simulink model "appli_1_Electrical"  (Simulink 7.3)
settings: Solver=ode23t  StartTime=0.0  StopTime=10.0  RelTol=1e-3
InitFcn:
  | R=10000;
  | C=1e-4;
StopFcn:
  | plot(1:length(signaux),signaux(:,1),1:length(signaux),signaux(:,2),1:length(signaux),signaux(:,3))
  |  axis([0 50 -0.2 1.2])
  | grid
  |  title('Tension théorique, d''entrée et charge de la capacité')
libraries: fl_lib x6, nesl_utility x3, elec_lib x1

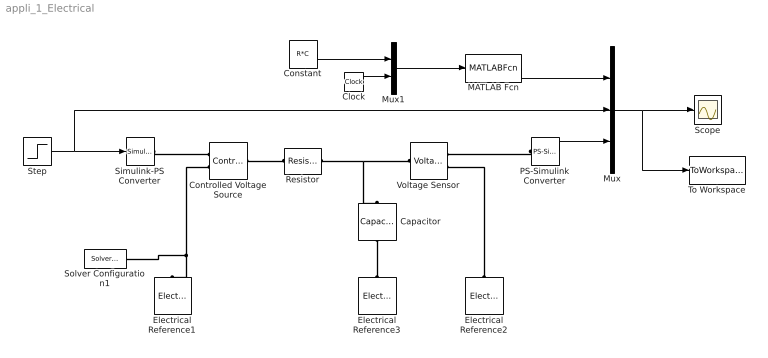
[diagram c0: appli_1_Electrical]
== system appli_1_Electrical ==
  Capacitor : fl_lib/Electrical/Electrical Elements/Capacitor  DialogController=NetworkEngine.DynNeDlgSource  SystemSampleTime=-1  c=C F  v0=0 V  r=0 Ohm  g=0 1/Ohm  i_Log=off  v_Log=off  vc_Log=off  LocalVarNames=|i|v|vc  LocalVarDescs=|i|v|Internal variable for voltage across capacitor term  LocalVarLogging=[0 0 0]
  Clock : Clock
  Constant : Constant  Value=R*C  OutDataType=fixdt(1, 16)  OutScaling=2^0
  Controlled Voltage Source : fl_lib/Electrical/Electrical Sources/Controlled Voltage Source  DialogController=NetworkEngine.DynNeDlgSource  SystemSampleTime=-1  i_Log=off  v_Log=off  LocalVarNames=|current|voltage|power  LocalVarDescs=|Current (A)|Voltage (V)|Power (W)  LocalVarLogging=[0 0 0]
  Electrical Reference1 : fl_lib/Electrical/Electrical Elements/Electrical Reference  DialogController=NetworkEngine.DynNeDlgSource  SystemSampleTime=-1  i_Log=off  LocalVarNames=|i  LocalVarDescs=|i  LocalVarLogging=0
  Electrical Reference2 : fl_lib/Electrical/Electrical Elements/Electrical Reference  DialogController=NetworkEngine.DynNeDlgSource  SystemSampleTime=-1  i_Log=off  LocalVarNames=|i  LocalVarDescs=|i  LocalVarLogging=0
  Electrical Reference3 : fl_lib/Electrical/Electrical Elements/Electrical Reference  DialogController=NetworkEngine.DynNeDlgSource  SystemSampleTime=-1  i_Log=off  LocalVarNames=|i  LocalVarDescs=|i  LocalVarLogging=0
  MATLAB Fcn : MATLABFcn  MATLABFcn=1-exp(-u(2)/u(1))
  Mux : Mux  Inputs=3
  Mux1 : Mux  Inputs=2
  PS-Simulink Converter : nesl_utility/PS-Simulink Converter  DialogController=NetworkEngine.DynNeUtilDlgSource  SystemSampleTime=-1  PhysicalDomain=network_engine_domain  LeftPortType=input  RightPortType=output  SubClassName=ps_output  Unit=1  AffineConversion=off
  Resistor : elec_lib/Passive Devices/Resistor  DialogController=NetworkEngine.DynNeDlgSource  SystemSampleTime=-1  SCALE=1  R_param=1  R=R Ohm  RSH=0 Ohm  LENGTH=1e-06 m  WIDTH=1e-06 m  NARROW=0 m  T_param=1  TC1=0 1/K  TC2=0 1/K^2  TOFFSET=0 K  TFIXED=300.15 K  TMEAS=300.15 K  LocalVarLogging=[]
  Scope : Scope
  Simulink-PS Converter : nesl_utility/Simulink-PS Converter  DialogController=NetworkEngine.DynNeUtilDlgSource  SystemSampleTime=-1  PhysicalDomain=network_engine_domain  LeftPortType=input  RightPortType=output  SubClassName=ps_input  Unit=1  AffineConversion=off  InputFilterTimeConstant=.001  UdotUserProvided=0
  Solver Configuration1 : nesl_utility/Solver Configuration  DialogController=NetworkEngine.DynNeUtilDlgSource  SystemSampleTime=-1  PhysicalDomain=network_engine_domain  LeftPortType=input  RightPortType=generic  SubClassName=solver  Accelerate=off  Profile=off  ResidualTolerance=1e-9  MaxNonlinIter=12  MaxModeIter=2  DoFixedCost=off  DoDC=off  LinearAlgebra=Sparse
  Step : Step  Time=0  SampleTime=0
  To Workspace : ToWorkspace  VariableName=signaux  SampleTime=-1  SaveFormat=Array
  Voltage Sensor : fl_lib/Electrical/Electrical Sensors/Voltage Sensor  DialogController=NetworkEngine.DynNeDlgSource  SystemSampleTime=-1  i1_Log=off  v1_Log=off  LocalVarNames=|i1|v1  LocalVarDescs=|i1|v1  LocalVarLogging=[]
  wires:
  Step/1 -> Simulink-PS Converter/1, Mux/2
  Mux/1 -> Scope/1, To Workspace/1
  Clock/1 -> Mux1/2
  Constant/1 -> Mux1/1
  Mux1/1 -> MATLAB Fcn/1
  PS-Simulink Converter/1 -> Mux/3
  MATLAB Fcn/1 -> Mux/1
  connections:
  Resistor/RConn1 -- Capacitor/LConn1 -- Voltage Sensor/LConn1
  Simulink-PS Converter/RConn1 -- Controlled Voltage Source/RConn1
  Controlled Voltage Source/RConn2 -- Electrical Reference1/LConn1 -- Solver Configuration1/RConn1
  Resistor/LConn1 -- Controlled Voltage Source/LConn1
  PS-Simulink Converter/LConn1 -- Voltage Sensor/RConn1
  Electrical Reference2/LConn1 -- Voltage Sensor/RConn2
  Electrical Reference3/LConn1 -- Capacitor/RConn1
